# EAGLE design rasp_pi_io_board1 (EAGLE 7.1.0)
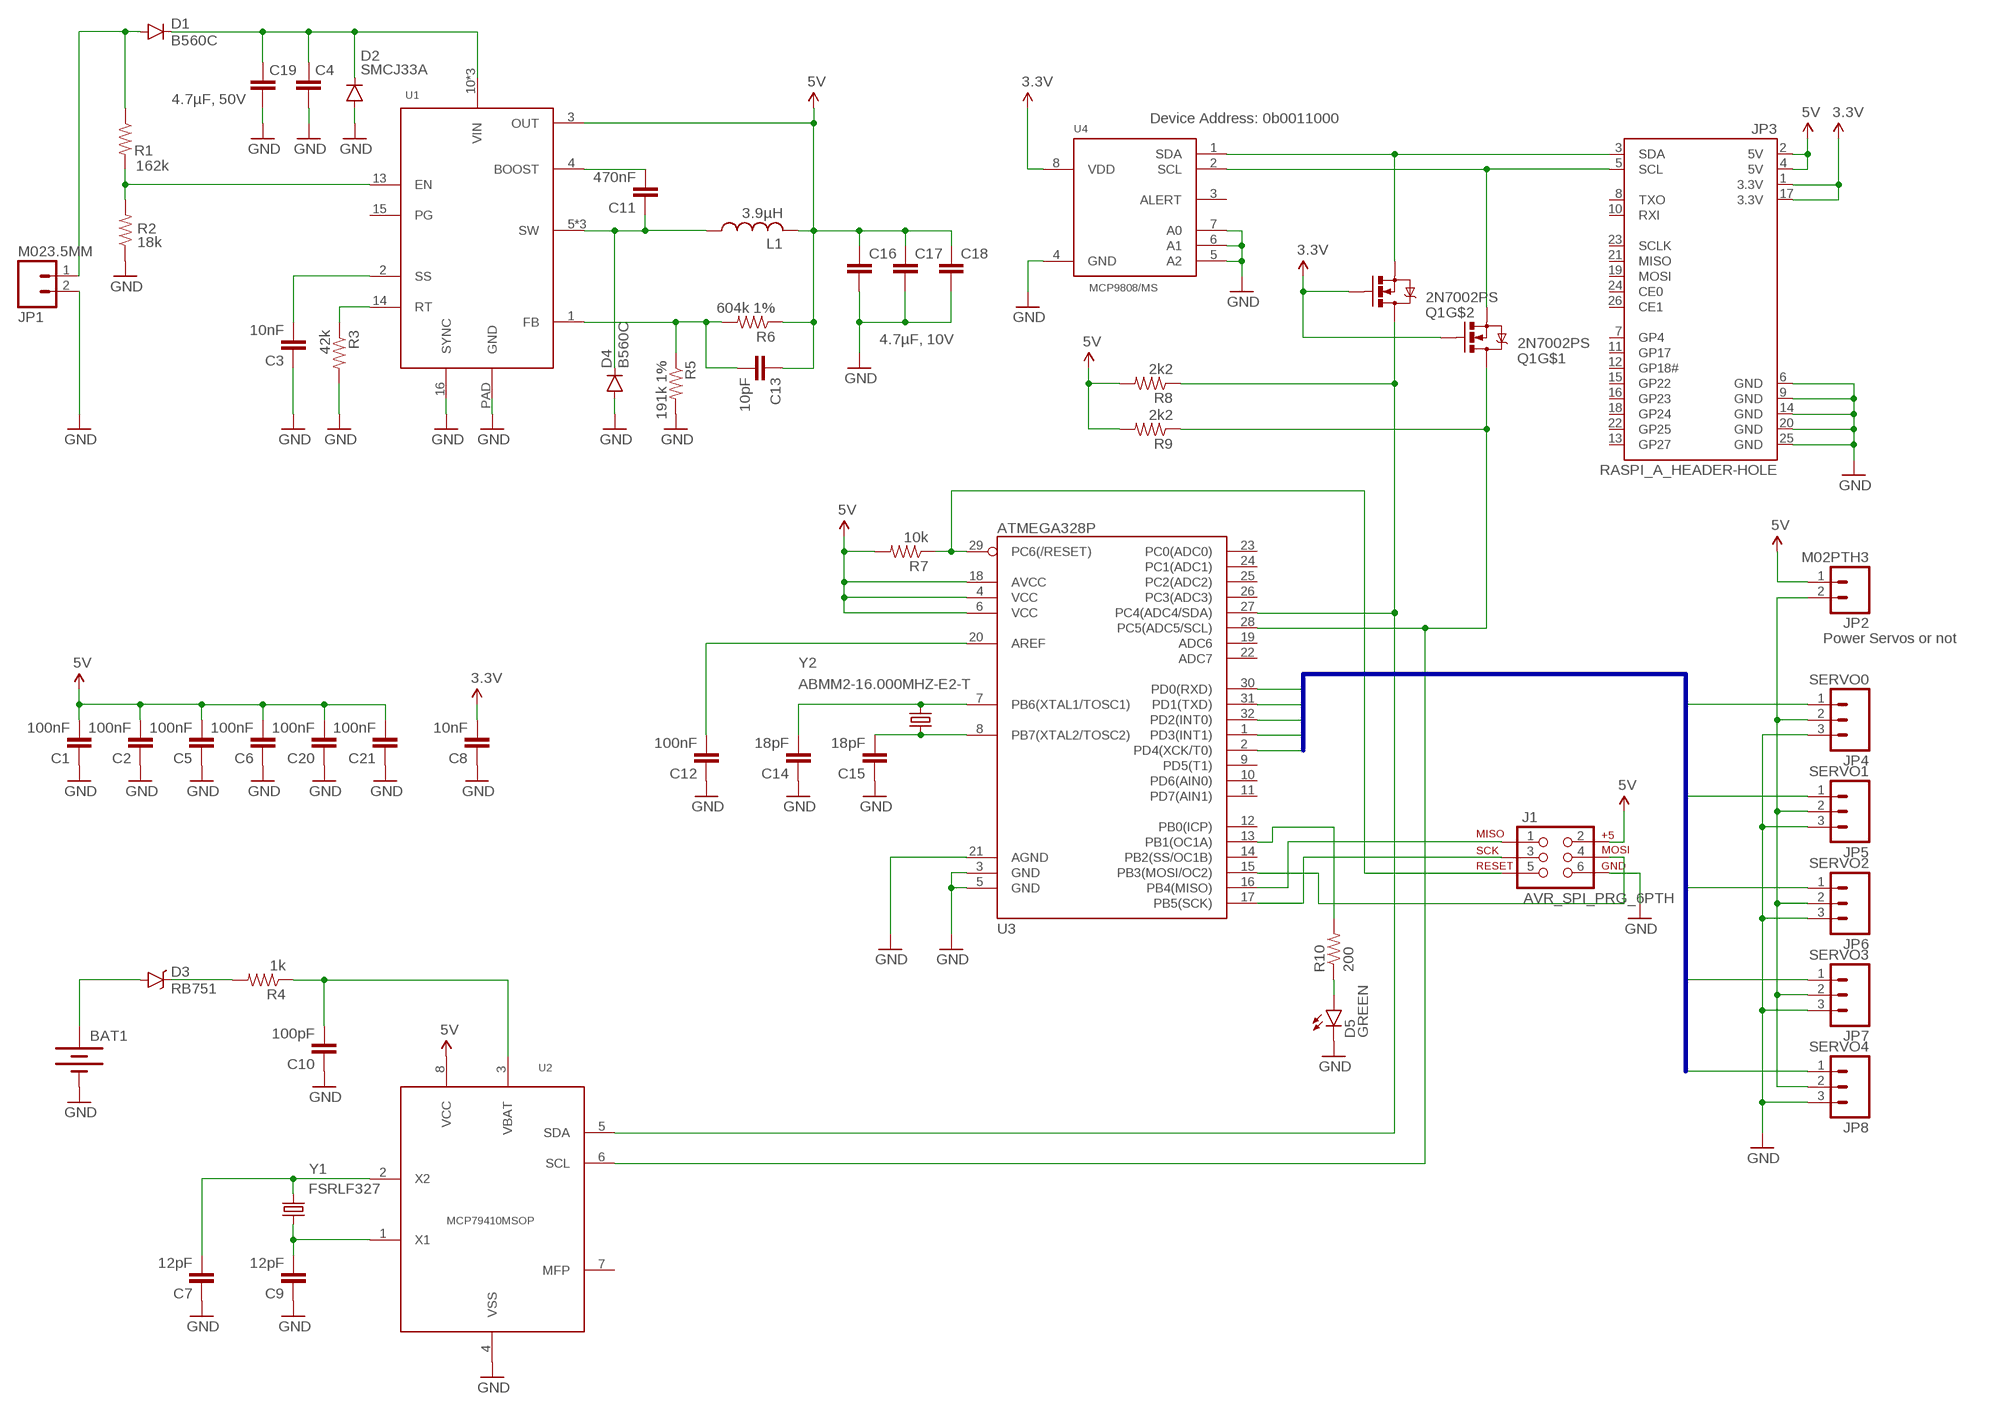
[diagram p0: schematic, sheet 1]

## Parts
BAT1  BATTERY20PTH  [BATTCOM_20MM_PTH]
C1  100nF  CAP0805  [0805]
C2  100nF  CAP0805  [0805]
C3  10nF  CAP0805  [0805]
C4  4.7µF, 50V  CAP1210  [1210]
C5  100nF  CAP0805  [0805]
C6  100nF  CAP0805  [0805]
C7  12pF  CAP0805  [0805]
C8  10nF  CAP0805  [0805]
C9  12pF  CAP0805  [0805]
C10  100pF  CAP0805  [0805]
C11  470nF  CAP0805  [0805]
C12  100nF  CAP0805  [0805]
C13  10pF  CAP0805  [0805]
C14  18pF  CAP0805  [0805]
C15  18pF  CAP0805  [0805]
C16  4.7µF, 10V  CAP1210  [1210]
C17  4.7µF, 10V  CAP1210  [1210]
C18  4.7µF, 10V  CAP1210  [1210]
C19  4.7µF, 50V  CAP1210  [1210]
C20  100nF  CAP0805  [0805]
C21  100nF  CAP0805  [0805]
D1  B560C  DIODESMC/DO-214AB  [SMC]
D2  SMCJ33A  DIODESMC/DO-214AB  [SMC]
D3  RB751  DIODE-SCHOTTKY-RB751  [SOD-523]
D4  B560C  DIODESMC/DO-214AB  [SMC]
D5  GREEN  LED-GREENLARGE  [LED-1206]
J1  AVR_SPI_PRG_6PTH  [2X3]
JP1  M023.5MM  [SCREWTERMINAL-3.5MM-2]
JP2  M02PTH3  [1X02_LONGPADS]
JP3  RASPI_A_HEADER-HOLE  [RASPI_A_GPIO_HEADER_HOLE]
JP4  SERVO0  M03LONGPADS  [1X03_LONGPADS]
JP5  SERVO1  M03LONGPADS  [1X03_LONGPADS]
JP6  SERVO2  M03LONGPADS  [1X03_LONGPADS]
JP7  SERVO3  M03LONGPADS  [1X03_LONGPADS]
JP8  SERVO4  M03LONGPADS  [1X03_LONGPADS]
L1  3.9µH  SRR1240_SERIES_INDUCTORS  [SRR1240_SERIES]
Q1  2N7002PS  [SOT363]
R1  162k  RESISTOR0805-RES  [0805]
R2  18k  RESISTOR0805-RES  [0805]
R3  42k  RESISTOR0805-RES  [0805]
R4  1k  RESISTOR0805-RES  [0805]
R5  191k 1%  RESISTOR0805-RES  [0805]
R6  604k 1%  RESISTOR0805-RES  [0805]
R7  10k  RESISTOR0805-RES  [0805]
R8  2k2  RESISTOR0805-RES  [0805]
R9  2k2  RESISTOR0805-RES  [0805]
R10  200  RESISTOR0805-RES  [0805]
U1  LT3995MSOP-16  [MSOP-16_EP]
U2  MCP79410MSOP  [MSOP-8]
U3  ATMEGA328P  ATMEGA328_SMT  [TQFP32-08]
U4  MCP9808/MS  [MSOP-8]
Y1  FSRLF327  [FSRLF327]
Y2  ABMM2-16.000MHZ-E2-T  ABMM2_SERIES  [ABMM2_SERIES]

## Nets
3.3V: C8.2 JP3.1(3.3V) JP3.17(3.3V) Q1.P$2(G1) Q1.P$5(G1) U4.8(VDD)
5V: C1.2 C2.2 C5.2 C6.2 C13.1 C16.1 C17.1 C18.1 C20.2 C21.2 J1.2 JP2.1 JP3.2(5V) JP3.4(5V) L1.P$2 R6.1 R7.2 R8.2 R9.2 U1.3(OUT) U2.8(VCC) U3.4(VCC) U3.6(VCC) U3.18(AVCC)
GND: BAT1.2(-) C1.1 C2.1 C3.1 C4.2 C5.1 C6.1 C7.1 C8.1 C9.1 C10.1 C12.1 C14.1 C15.1 C16.2 C17.2 C18.2 C19.2 C20.1 C21.1 D2.A D4.A D5.C J1.6 JP1.2 JP3.6(GND) JP3.9(GND) JP3.14(GND) JP3.20(GND) JP3.25(GND) JP4.3 JP5.3 JP6.3 JP7.3 JP8.3 R2.1 R3.2 R5.2 U1.16(SYNC) U1.PAD(GND) U2.4(VSS) U3.3(GND) U3.5(GND) U3.21(AGND) U4.4(GND) U4.5(A2) U4.6(A1) U4.7(A0)
N$1: C14.2 U3.7(PB6(XTAL1/TOSC1)) Y2.P$3
N$2: C15.2 U3.8(PB7(XTAL2/TOSC2)) Y2.P$1
N$3: D1.A JP1.1 R1.1
N$4: R1.2 R2.2 U1.13(EN)
N$5: R3.1 U1.14(RT)
N$6: J1.5 R7.1 U3.29(PC6(/RESET))
N$7: C11.2 U1.4(BOOST)
N$8: C11.1 D4.C L1.P$1 U1.5(SW) U1.6(SW) U1.7(SW)
N$9: C12.2 U3.20(AREF)
N$10: J1.3 U3.17(PB5(SCK))
N$11: J1.1 U3.16(PB4(MISO))
N$12: J1.4 U3.15(PB3(MOSI/OC2))
N$13: D5.A R10.1
N$14: R10.2 U3.13(PB1(OC1A))
N$15: JP3.3(SDA) Q1.P$4(S1) U4.1(SDA)
N$16: JP3.5(SCL) Q1.P$1(S1) U4.2(SCL)
N$17: Q1.P$3(D1) R8.1 U2.5(SDA) U3.27(PC4(ADC4/SDA))
N$18: Q1.P$6(D1) R9.1 U2.6(SCL) U3.28(PC5(ADC5/SCL))
N$19: C13.2 R5.1 R6.2 U1.1(FB)
N$20: C4.1 C19.1 D1.C D2.C U1.10(VIN) U1.11(VIN) U1.12(VIN)
N$21: C3.2 U1.2(SS)
N$22: JP2.2 JP4.2 JP5.2 JP6.2 JP7.2 JP8.2
N$23: C10.2 R4.1 U2.3(VBAT)
N$24: C9.2 U2.1(X1) Y1.P$4
N$25: C7.2 U2.2(X2) Y1.P$1
N$26: D3.C R4.2
N$27: BAT1.1(+) D3.A
PD0: JP4.1 U3.30(PD0(RXD))
PD1: JP5.1 U3.31(PD1(TXD))
PD2: JP6.1 U3.32(PD2(INT0))
PD3: JP7.1 U3.1(PD3(INT1))
PD4: JP8.1 U3.2(PD4(XCK/T0))
Unconnected: JP3.7(GP4) JP3.8(TXO) JP3.10(RXI) JP3.11(GP17) JP3.12(GP18#) JP3.13(GP27) JP3.15(GP22) JP3.16(GP23) JP3.18(GP24) JP3.19(MOSI) JP3.21(MISO) JP3.22(GP25) JP3.23(SCLK) JP3.24(CE0) JP3.26(CE1) U1.15(PG) U2.7(MFP) U3.9(PD5(T1)) U3.10(PD6(AIN0)) U3.11(PD7(AIN1)) U3.12(PB0(ICP)) U3.14(PB2(SS/OC1B)) U3.19(ADC6) U3.22(ADC7) U3.23(PC0(ADC0)) U3.24(PC1(ADC1)) U3.25(PC2(ADC2)) U3.26(PC3(ADC3)) U4.3(ALERT)

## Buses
PD[0..7]

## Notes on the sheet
- Device Address: 0b0011000
- Power Servos or not

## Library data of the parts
BAT1 = SparkFun-Electromechanical:BATTERY: Battery Holders; FARNELL: 1339839
C1 C2 C5 C6 C12 C20 C21 = SparkFun-Capacitors:CAP: Capacitor; FARNELL: 7569564
C3 C8 = SparkFun-Capacitors:CAP: Capacitor; FARNELL: 1650952
C4 C19 = SparkFun-Passives:CAP: Capacitor; FARNELL: 2211158
C7 C9 = SparkFun-Capacitors:CAP: Capacitor; FARNELL: 2218857
C10 = SparkFun-Capacitors:CAP: Capacitor; FARNELL: 1855317
C11 = SparkFun-Capacitors:CAP: Capacitor; FARNELL: 2210986
C13 = SparkFun-Capacitors:CAP: Capacitor; FARNELL: 2219447
C14 C15 = SparkFun-Passives:CAP: Capacitor; FARNELL: 2218861
C16-C18 = SparkFun-Passives:CAP: Capacitor; FARNELL: 2113075
D1 D4 = SparkFun-DiscreteSemi:DIODE: Diode; FARNELL: 1858602
D2 = SparkFun-DiscreteSemi:DIODE: Diode; FARNELL: 1827624
D3 = SparkFun-DiscreteSemi:DIODE-SCHOTTKY: Schottky diodes in SFE's production catalog; FARNELL: 2317437; PROD_ID: DIO-11018
D5 = SparkFun-LED:LED-GREEN: Various green LEDs; FARNELL: 2099247; PROD_ID: DIO-00862
J1 = SparkFun-Connectors:AVR_SPI_PRG_6: AVR ISP 6 Pin This is the reduced ISP connector for AVR programming. Common on Arduino. This footprint will take up less PCB space and can be used with a 10-pin to 6-pin adapter such as SKU: BOB-08508 **Special note about "TEST_POINT" package. The stop mask is on the top side, so if you want your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; FARNELL: 2381222
JP1 JP2 = SparkFun-Connectors:M02: Standard 2-pin 0.1" header. Use with
JP3 = det_lib:RASPI_A_HEADER: Raspberry Pi A Header; FARNELL: 9138650
JP4-JP8 = SparkFun-Connectors:M03: Header 3 Standard 3-pin 0.1" header. Use with straight break away headers (SKU : PRT-00116), right angle break away headers (PRT-00553), swiss pins (PRT-00743), machine pins (PRT-00117), and female headers (PRT-00115). Molex polarized connector foot print use with SKU : PRT-08232 with associated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
L1 = det_lib:SRR1240_SERIES_INDUCTORS: Inductor; FARNELL: 2333737
Q1 = det_lib:2N7002PS: 2N7002PS Dual 2N7002 mosfets in SOT363 package.; FARNELL: 1859846
R1 = SparkFun-Resistors:RESISTOR: Resistor; FARNELL: 1810721
R2 = SparkFun-Resistors:RESISTOR: Resistor; FARNELL: 1688507RL
R3 = SparkFun-Resistors:RESISTOR: Resistor; FARNELL: 2141879
R4 = SparkFun-Resistors:RESISTOR: Resistor; FARNELL: 1653280
R5 = SparkFun-Resistors:RESISTOR: Resistor; FARNELL: 2117405
R6 = SparkFun-Resistors:RESISTOR: Resistor; FARNELL: 1653024
R7 = SparkFun-Resistors:RESISTOR: Resistor; FARNELL: 1612522
R8 R9 = SparkFun-Resistors:RESISTOR: Resistor; FARNELL: 2082065
R10 = SparkFun-Resistors:RESISTOR: Resistor; FARNELL: 1577649
U1 = det_lib:LT3995: LT3995 Step-Down Switching Regulator Buck converter.; FARNELL: 2356021
U2 = det_lib:MCP79410: Real-time clock; FARNELL: 1823153
U3 = SparkFun-DigitalIC:ATMEGA328_SMT: 32-Pin Atmega328 part Commonly used on Arduino compatible boards Available in QFP and QFN packages TQFP is IC-09069 QFN is non-stock; FARNELL: 1715486; PROD_ID: IC-09069
U4 = det_lib:MCP9808: MCP9808 ±0.5°C Maximum Accuracy Digital Temperature Sensor I2C temperature sensor with ±0.5°C maximum accuracy.; FARNELL: 2080523
Y1 = det_lib:FSRLF327: Crystal; FARNELL: 2064035
Y2 = det_lib:ABMM2_SERIES: Crystal; FARNELL: 2101343

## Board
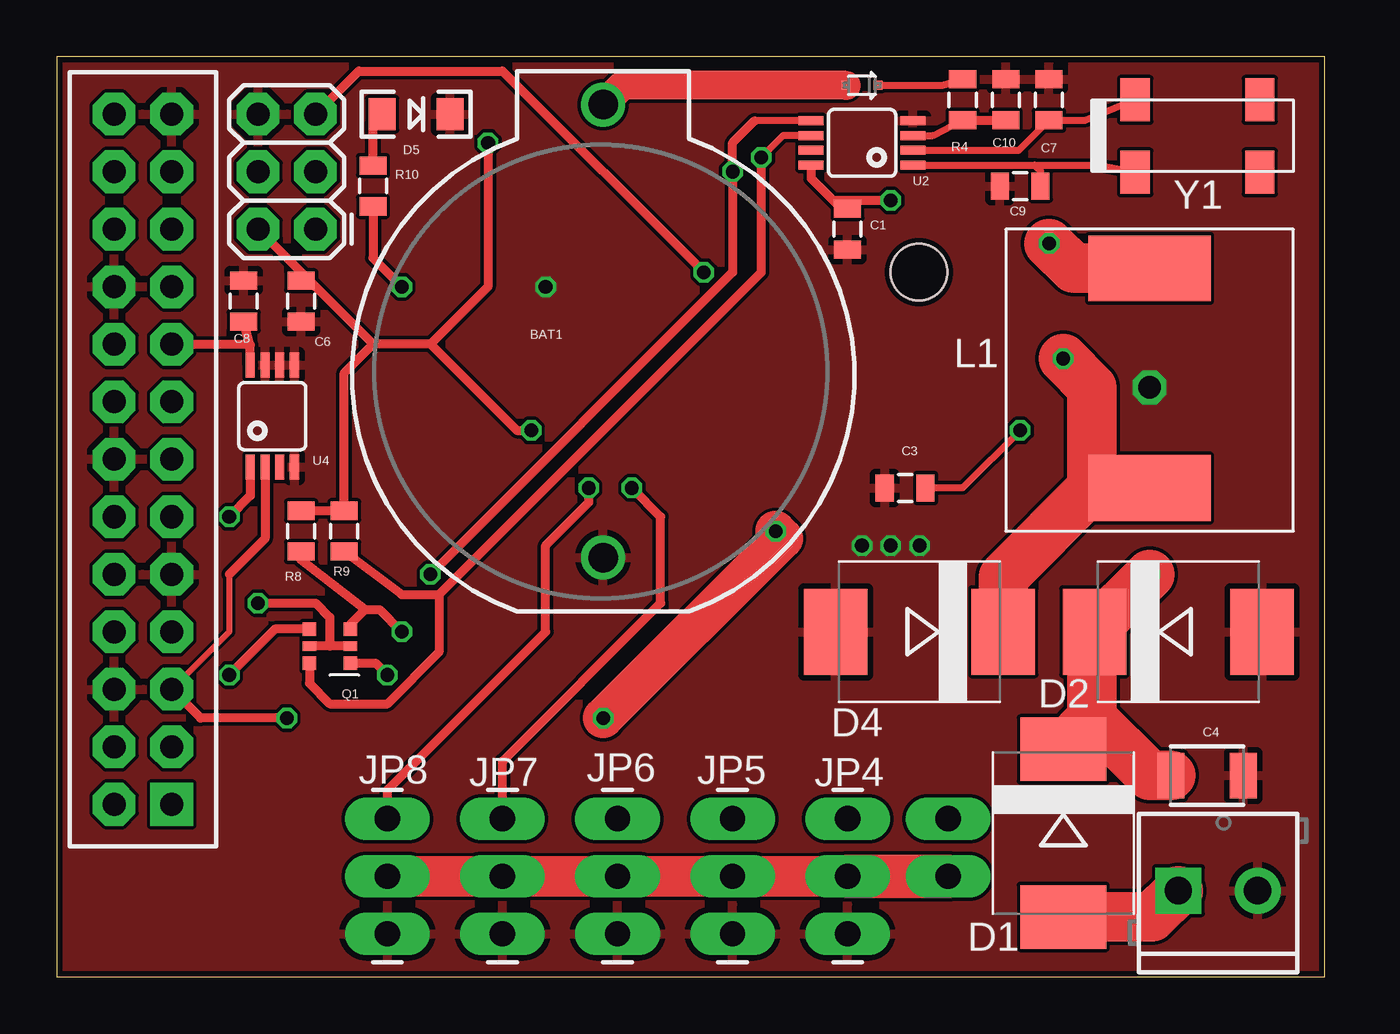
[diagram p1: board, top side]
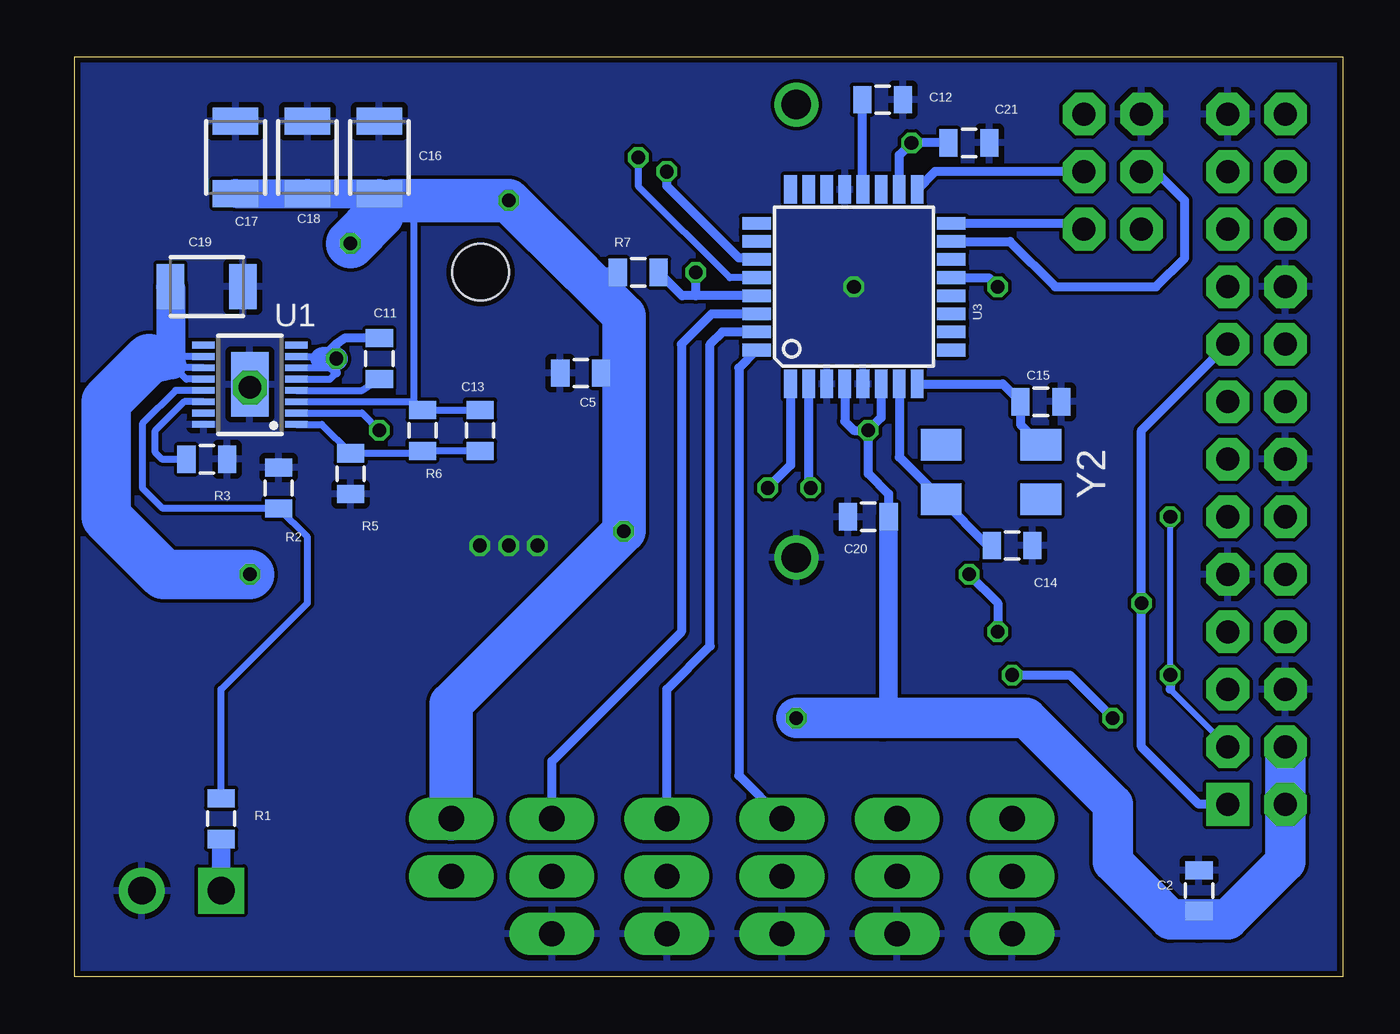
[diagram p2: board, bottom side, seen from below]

Size 56 x 40.63 mm. Coordinates in mm from the lower left corner, seen from the top.
Outline: 0,0 56,0 56,40.63 0,40.63 0,0
Copper layers (1*16): Top 0.035mm / dielectric 1.5mm / Bottom 0.035mm
Design rules "SeeedStudio_2layer_DRU_no_angle_20140221": minimum track width 6mil, minimum drill 12mil, track to track 6mil, track to pad 6mil, pad to pad 6mil, via to via 6mil, smd to smd 0mil, copper to edge 10mil, drill to drill 10mil, minimum pad ring 10mil, minimum via ring 6mil, stop-mask expansion 2mil, vias tented up to drill 100mil, thermal gap 10mil

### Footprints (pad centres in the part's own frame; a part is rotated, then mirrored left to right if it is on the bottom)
BATTCOM_20MM_PTH = drill 1.3: 1 11.85,0; 2 -8.15,0
0805 = smd 0.8 x 1.2: 1 -0.9,0; 2 0.9,0
1210 = smd 1.2 x 2: 1 -1.6,0; 2 1.6,0
SMC = smd 2.8 x 3.8: A 3.7,0; C -3.7,0
SOD-523 = smd 0.4 x 0.4: A -0.7,0; C 0.7,0
LED-1206 = smd 1.2 x 1.4: A -1.5,0; C 1.5,0
2X3 = drill 1.016 pad 1.88 octagon: 1 0,0; 2 0,2.54; 3 2.54,0; 4 2.54,2.54; 5 5.08,0; 6 5.08,2.54
SCREWTERMINAL-3.5MM-2 = drill 1.2 pad 2.032 square: 1 0,0 | drill 1.2 pad 2.032: 2 3.5,0
1X02_LONGPADS = drill 1.118 pad 1.88 long: 1 0,0; 2 2.54,0
RASPI_A_GPIO_HEADER_HOLE = drill 1.016 pad 1.88 square: 1 0,0 | drill 1.016 pad 1.88 octagon: 2 -2.54,0; 3 0,2.54; 4 -2.54,2.54; 5 0,5.08; 6 -2.54,5.08; 7 0,7.62; 8 -2.54,7.62; 9 0,10.16; 10 -2.54,10.16; 11 0,12.7; 12 -2.54,12.7; 13 0,15.24; 14 -2.54,15.24; 15 0,17.78; 16 -2.54,17.78; 17 0,20.32; 18 -2.54,20.32; 19 0,22.86; 20 -2.54,22.86; 21 0,25.4; 22 -2.54,25.4; 23 0,27.94; 24 -2.54,27.94; 25 0,30.48; 26 -2.54,30.48 | hole 2.5: 33,23.5
1X03_LONGPADS = drill 1.118 pad 1.88 long: 1 0,0; 2 2.54,0; 3 5.08,0
SRR1240_SERIES = smd 2.9 x 5.4: P$1 0,0; P$2 9.7,0
SOT363 = smd 0.6 x 0.6: P$1 -0.9,0.75; P$3 -0.9,-0.75; P$4 0.9,-0.75; P$6 0.9,0.75 | smd 0.6 x 0.4: P$2 -0.9,0; P$5 0.9,0
MSOP-16_EP = smd 0.3 x 1: 1 -1,0.49; 2 -0.5,0.49; 3 0,0.49; 4 0.5,0.49; 5 1,0.49; 6 1.5,0.49; 7 2,0.49; 8 2.5,0.49; 9 2.5,4.59; 10 2,4.59; 11 1.5,4.59; 12 1,4.59; 13 0.5,4.59; 14 0,4.59; 15 -0.5,4.59; 16 -1,4.59 | smd 2.845 x 1.651: PAD 0.76,2.54
MSOP-8 = smd 0.4 x 1.1: 1 -0.975,-2.25; 2 -0.325,-2.25; 3 0.325,-2.25; 4 0.975,-2.25; 5 0.975,2.25; 6 0.325,2.25; 7 -0.325,2.25; 8 -0.975,2.25
TQFP32-08 = smd 1.27 x 0.559: 1 -4.293,2.8; 2 -4.293,2; 3 -4.293,1.2; 4 -4.293,0.4; 5 -4.293,-0.4; 6 -4.293,-1.2; 7 -4.293,-2; 8 -4.293,-2.8; 17 4.293,-2.8; 18 4.293,-2; 19 4.293,-1.2; 20 4.293,-0.4; 21 4.293,0.4; 22 4.293,1.2; 23 4.293,2; 24 4.293,2.8 | smd 0.559 x 1.27: 9 -2.8,-4.293; 10 -2,-4.293; 11 -1.2,-4.293; 12 -0.4,-4.293; 13 0.4,-4.293; 14 1.2,-4.293; 15 2,-4.293; 16 2.8,-4.293; 25 2.8,4.293; 26 2,4.293; 27 1.2,4.293; 28 0.4,4.293; 29 -0.4,4.293; 30 -1.2,4.293; 31 -2,4.293; 32 -2.8,4.293
FSRLF327 = smd 1.3 x 1.9: P$1 0,0; P$2 5.5,0; P$3 5.5,-3.2; P$4 0,-3.2
ABMM2_SERIES = smd 1.8 x 1.4: P$1 0,0; P$2 4.4,0; P$3 4.4,2.4; P$4 0,2.4

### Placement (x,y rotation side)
BAT1  24.13,26.67 90 top
C1  34.92,33.02 90 top
C2  6.35,3.81 270 bottom
C3  37.47,21.59 0 top
C4  50.8,8.89 0 top
C5  33.66,26.67 0 bottom
C6  10.79,29.84 90 top
C7  43.81,38.73 270 top
C8  8.26,29.84 270 top
C9  42.55,34.92 0 top
C10  41.91,38.73 270 top
C11  42.55,27.3 270 bottom
C12  20.32,38.73 180 bottom
C13  38.1,24.13 270 bottom
C14  14.61,19.05 180 bottom
C15  13.34,25.4 180 bottom
C16  42.55,36.2 90 bottom
C17  48.9,36.2 90 bottom
C18  45.72,36.2 90 bottom
C19  50.16,30.48 0 bottom
C20  20.95,20.32 0 bottom
C21  16.51,36.83 180 bottom
D1  44.45,6.35 270 top
D2  49.53,15.24 0 top
D3  35.56,39.37 0 top
D4  38.1,15.24 180 top
D5  15.88,38.1 0 top
J1  11.43,33.02 90 top
JP1  49.53,3.81 0 top
JP2  39.37,6.99 270 top
JP3  5.08,7.62 0 top
JP4  34.92,6.99 270 top
JP5  29.84,6.99 270 top
JP6  24.77,6.99 270 top
JP7  19.68,6.99 270 top
JP8  14.61,6.99 270 top
L1  48.26,21.59 90 top
Q1  12.06,14.61 180 top
R1  49.53,6.99 90 bottom
R2  46.99,21.59 270 bottom
R3  50.16,22.86 0 bottom
R4  40.01,38.73 90 top
R5  43.81,22.23 270 bottom
R6  40.64,24.13 270 bottom
R7  31.11,31.11 180 bottom
R8  10.79,19.68 90 top
R9  12.7,19.68 90 top
R10  13.97,34.92 270 top
U1  45.72,25.4 90 bottom
U2  35.56,36.83 90 top
U3  21.59,30.48 90 bottom
U4  9.53,24.77 0 top
Y1  47.62,38.73 0 top
Y2  13.34,23.5 180 bottom

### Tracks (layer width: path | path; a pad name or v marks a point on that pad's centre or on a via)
3.3V  (via drill 0.6)
  Top 0.406: JP3.17 8.52,27.94 | 8.52,27.94 C8.2 | Q1.P$2 12.06,14.61 | 12.06,14.61 Q1.P$5 | v8.89,16.51 11.43,16.51 12.06,15.88 12.06,14.61 | U4.8 8.55,27.91 8.52,27.94
  Bottom 0.406: JP3.1 6.35,7.62 8.89,10.16 v8.89,16.51 8.89,24.13 JP3.17
5V  (via drill 0.6)
  Top 0.406: v19.05,36.83 19.05,30.48 16.51,27.94 | 16.51,27.94 13.97,27.94 | 13.97,27.94 11.43,30.48 | 11.43,30.48 J1.2 | v36.83,34.29 34.29,34.29 | U2.8 33.31,35.27 34.29,34.29 | R8.2 R9.2 12.7,26.67 13.97,27.94 | C1.2 34.66,33.92 34.29,34.29 | 16.51,27.94 20.32,24.13 v20.95,24.13 | C6.2 11.43,30.48
  Top 1.778: v24.13,11.43 32.07,19.37 v31.75,19.68
  Top 2.184: L1.P$2 44.91,31.29 v43.81,32.38
  Bottom 0.305: U1.3 41.01,25.4 | C13.1 R6.1 41.01,25.4 | 41.01,25.4 41.01,33.39 41.91,34.29 42.24,34.29 C16.1
  Bottom 0.406: U3.4 21.99,24.53 21.59,24.13 v20.95,24.13 | U3.6 20.39,24.7 v20.95,24.13 | U3.18 19.59,36.29 v19.05,36.83 C21.2 | R7.2 33.66,31.11 | C5.2 31.75,26.67 | v20.95,24.13 20.95,22.23 20.05,21.32 C20.2
  Bottom 0.813: C20.2 20.05,11.7 20.32,11.43
  Bottom 1.016: C2.2 6.35,2.54
  Bottom 1.27: C17.1 C18.1 C16.1 42.55,33.66
  Bottom 1.778: v24.13,11.43 20.32,11.43 13.97,11.43 10.16,7.62 10.16,5.08 7.62,2.54 6.35,2.54 5.08,2.54 2.54,5.08 JP3.2 JP3.4
  Bottom 1.93: JP2.1 39.37,12.06 v31.75,19.68 31.75,26.67 31.75,29.21 33.66,31.11 v36.83,34.29 41.91,34.29
  Bottom 2.184: v43.81,32.38 42.55,33.66
GND  (via drill 0.6, 1)
  Bottom 0.406: v48.26,26.04 U1.PAD
  other vias: 35.56,19.05 36.83,19.05 38.1,19.05 21.59,30.48
  pour Top: -1.27,40.64 -1.27,0 105.41,0 105.41,40.64
  pour Bottom: 0,40.64 96.52,40.64 96.52,0 0,0
N$1
  Bottom 0.406: 17.41,20.77 Y2.P$3 | U3.7 19.59,22.95 Y2.P$3 | 18.15,20.68 Y2.P$3 | C14.2 15.69,19.05 Y2.P$3
N$2
  Bottom 0.406: U3.8 15.02,26.19 C15.2 14.23,24.39 Y2.P$1
N$3
  Top 2.184: D1.A 48.37,2.65 JP1.1
  Bottom 0.813: R1.1 JP1.1
N$4
  Bottom 0.305: U1.13 51.55,25.9 53.01,24.43 53.01,21.59 52.11,20.69 R2.2 45.72,19.42 45.72,16.51 49.53,12.7 R1.2
N$5
  Bottom 0.305: U1.14 51.16,25.4 52.46,24.09 52.46,23.18 52.16,22.88 51.08,22.88 R3.1
N$6  (via drill 0.6)
  Top 0.406: J1.5 13.34,40.01 19.68,40.01 v28.57,31.11
  Bottom 0.406: U3.29 28.57,30.08 | 28.57,30.08 29.18,30.08 R7.1 | v28.57,31.11 28.57,30.08
N$7
  Bottom 0.305: U1.4 43.31,25.9 C11.2
N$8  (via drill 0.6)
  Top 2.184: D4.C 41.8,17.67 45.72,21.59 | L1.P$1 45.72,21.59 | 45.72,21.59 45.72,26.04 v44.45,27.3
  Bottom 0.305: U1.7 44.99,27.4 | U1.5 44.72,26.4 44.45,26.67 | U1.6 44.68,26.9
  Bottom 0.406: 44.99,27.4 44.45,27.94 | 44.45,27.94 v44.45,27.3 44.45,26.67 44.68,26.9 | C11.1 44.08,28.2 44.45,27.94
  Bottom 1.016: v44.45,27.3 45.09,27.3
N$9
  Bottom 0.406: U3.20 21.22,34.77 C12.2
N$10
  Bottom 0.406: J1.3 18,35.56 U3.17
N$11
  Bottom 0.406: U3.16 11.69,33.28 J1.1
N$12
  Bottom 0.406: U3.15 14.7,32.48 12.7,30.48 8.26,30.48 6.99,31.75 6.99,34.29 8.26,35.56 J1.4
N$13
  Top 0.406: R10.1 13.97,37.7 D5.A
N$14  (via drill 0.6)
  Top 0.406: R10.2 13.97,31.75 v15.24,30.48
  Bottom 0.406: U3.13 15.64,30.88 v15.24,30.48
N$15  (via drill 0.6)
  Top 0.406: Q1.P$4 9.64,15.36 v7.62,13.34 | U4.1 8.55,21.25 v7.62,20.32
  Bottom 0.254: v7.62,13.34 v7.62,20.32 | JP3.3 7.62,12.7
  Bottom 0.406: v7.62,13.34 7.62,12.7
N$16  (via drill 0.6)
  Top 0.254: JP3.5 7.62,15.24 7.62,17.78
  Top 0.406: Q1.P$1 14.09,13.86 v14.61,13.34 | v10.16,11.43 6.35,11.43 JP3.5 | U4.2 9.2,19.36 7.62,17.78
  Bottom 0.406: v14.61,13.34 12.06,13.34 v10.16,11.43
N$17  (via drill 0.6)
  Top 0.305: U2.5 30.82,37.8
  Top 0.406: 13.62,16.22 10.79,18.41 R8.1 | v16.51,17.78 29.84,31.11 v29.84,35.56 29.84,36.83 30.82,37.8 | 13.62,16.22 14.26,16.22 v15.24,15.24 | Q1.P$3 12.96,15.56 13.62,16.22
  Bottom 0.305: 25.95,31.75 U3.27
  Bottom 0.406: 25.95,31.75 26.67,31.75 29.84,34.92 v29.84,35.56 | v16.51,17.78 15.24,16.51 v15.24,15.24
N$18  (via drill 0.6)
  Top 0.305: U2.6 32.08,37.16 v31.11,36.2
  Top 0.406: 16.88,16.88 15.24,16.88 R9.1 | 16.88,16.88 31.11,31.11 v31.11,36.2 | 16.88,16.88 16.88,14.34 14.61,12.06 12.06,12.06 11.16,12.96 Q1.P$6
  Bottom 0.305: v31.11,36.2 31.11,34.92 27.07,30.88 U3.28
N$19
  Bottom 0.305: U1.1 45.09,24.4 R5.1 40.74,23.12 R6.2 C13.2
N$20  (via drill 0.6)
  Top 2.184: D1.C 44.45,10.16 45.72,11.43 | 45.72,11.43 45.72,15.13 D2.C 45.83,15.35 v48.26,17.78 | C4.1 48.26,8.89 45.72,11.43
  Bottom 0.305: U1.10 52.07,27.4 | U1.12 51.07,26.4 51.57,26.9 U1.11
  Bottom 0.406: 51.57,26.9 51.7,27.04 52.07,27.4
  Bottom 1.27: C19.1 51.77,27.09 51.7,27.04 53.34,26.67
  Bottom 2.184: v48.26,17.78 52.07,17.78 54.61,20.32 54.61,25.4 53.34,26.67 52.7,27.3
N$21  (via drill 0.6)
  Top 0.305: v42.55,24.13 40.01,21.59 C3.2
  Bottom 0.305: U1.2 43.31,24.9 v42.55,24.13
N$22
  Top 1.778: JP8.2 JP7.2 JP6.2 JP5.2 JP4.2
  Top 1.93: JP4.2 JP2.2
N$23
  Top 0.305: U2.3 38.69,37.16 R4.1
  Top 0.406: R4.1 C10.2
N$24
  Top 0.305: U2.1 43.18,35.85 | 43.18,35.85 46.03,35.85 Y1.P$4 | C9.2 43.45,35.59 43.18,35.85
N$25
  Top 0.305: U2.2 42.48,36.51 C7.2 45.45,37.84 Y1.P$1
N$26
  Top 0.305: D3.C 39.1,39.37 R4.2
N$27
  Top 1.27: D3.A 24.98,39.37 BAT1.1
PD0
  Bottom 0.406: U3.30 27.87,29.28 29.21,27.94 29.21,15.24 34.92,9.53 JP4.1
PD1
  Bottom 0.406: U3.31 27.4,28.48 27.94,27.94 27.94,14.61 29.84,12.7 JP5.1
PD2
  Bottom 0.406: JP6.1 26.67,8.89 26.67,26.89 U3.32
PD3  (via drill 0.6)
  Top 0.406: JP7.1 19.68,9.53 26.67,16.51 26.67,20.32 v25.4,21.59
  Bottom 0.406: U3.1 24.39,22.6 v25.4,21.59
PD4  (via drill 0.6)
  Top 0.406: v23.5,21.59 23.5,20.95 21.59,19.05 21.59,15.24 14.61,8.26 JP8.1
  Bottom 0.406: U3.2 23.59,21.68 v23.5,21.59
